(* Logix 5000 AddOnInstructionDefinition export YAI_Assy_155_118_EIP_Hz; software revision 21.03 *)

ADD_ON_INSTRUCTION YAI_Assy_155_118_EIP_Hz   (* revision 1.0, vendor Yaskawa America, Inc. *)
// YAI Assembly 155 and 118
// Help:
// This add-on instruction is for use with input assemblie 166 and output assemblies 116.
// Node_Input_Assy is defined as the node's input assembly integer array.
// Node_Output_Assy is defined as the node's output assembly integer array.
// Torque limit/reference, torque compensation and torque output variables are only available with A1000.
VAR_IN_OUT
   Node_Input_Assy : AB:ETHERNET_MODULE_INT_40Bytes:I:0; {required}   // Input assembly words
   Node_Output_Assy : AB:ETHERNET_MODULE_INT_12Bytes:O:0; {required}   // Output assembly words
END_VAR
VAR_INPUT
   RunFwd : BOOL; {visible}   // Forward run command
   RunRev : BOOL; {visible}   // Reverse run command
   MFI_3 : BOOL; {visible}   // Multi-function input 3
   MFI_4 : BOOL; {visible}   // Multi-function input 4
   MFI_5 : BOOL; {visible}   // Multi-function input 5
   MFI_6 : BOOL; {visible}   // Multi-function input 6
   MFI_7 : BOOL; {visible}   // Multi-function input 7
   MFI_8 : BOOL; {visible}   // Multi-function input 8
   External_Fault : BOOL;   // External fault command (EF0)
   FaultReset : BOOL; {visible}   // Fault reset command
   MFO_1 : BOOL; {visible}   // Multi-function output (M1-M2 for A/P1000, MA/MB/MC for V1000)
   MFO_2 : BOOL; {visible}   // Multi-function output (M3-M4 for A/P1000, P1 for V1000)
   MFO_3 : BOOL; {visible}   // Multi-function output (M5-M6 for A/P1000, P2 for V1000)
   Freq_Ref : REAL; {visible}   // Frequency reference command in Hz (xx.xx resolution)
   Digital_Output_Fault_Enable : BOOL;   // Bit to enable control of fault output relay over the network
END_VAR
VAR_OUTPUT
   Running : BOOL; {access Read Only, visible}   // Drive running forward status bit
   ZSP : BOOL; {access Read Only, visible}   // Drive zero speed status bit
   RunningRev : BOOL; {access Read Only, visible}   // Drive running reverse status bit
   Reset : BOOL; {access Read Only, visible}   // Drive reset command status bit
   At_Speed : BOOL; {access Read Only, visible}   // Drive at commanded speed status bit
   Ready : BOOL; {access Read Only, visible}   // Drive ready status bit
   Alarm : BOOL; {access Read Only, visible}   // Drive alarm status bit
   Faulted : BOOL; {access Read Only, visible}   // Drive faulted status bit
   OPE : BOOL; {access Read Only}   // OPE alarm/fault present
   UV : BOOL; {access Read Only}   // Drive in UV (undervoltage) state status bit
   NetCtrlStatus : BOOL; {access Read Only, visible}   // Drive network run source status bit (1 = source coming from network)
   MFO_1_Status : BOOL; {access Read Only, visible}   // Drive multi-function output 1 (M1-M2 for A/P1000, MA/MB/MC for V1000) status
   MFO_2_Status : BOOL; {access Read Only, visible}   // Drive multi-function output 1 (M3-M4 for A/P1000, P1 for V1000) status
   MFO_3_Status : BOOL; {access Read Only, visible}   // Drive multi-function output 1 (M5-M6 for A/P1000, P2 for V1000) status
   ZSV : BOOL; {access Read Only, visible}   // Drive zero servo completed status bit
   Motor_Speed : REAL; {access Read Only, visible}   // Motor speed in Hz (xx.xx resolution)
   Torque_Actual : REAL; {access Read Only, visible}   // Drive torque output in % (xxx.x resolution)
   PG1_Count : INT; {access Read Only}   // Encoder feedback count
   Freq_Cmd : REAL; {access Read Only, visible}   // Commanded frequency in Hz (xx.xx resolution)
   Output_Freq : REAL; {access Read Only, visible}   // Drive output frequency in Hz (xx.xx resolution)
   Output_Current : REAL; {access Read Only, visible}   // Drive output current in A (xxx.x resolution)
   Analog_Input_1_Level : REAL; {access Read Only}   // Analog input 1 level in % (xxx.x resolution)
   DC_Bus_Volt : INT; {access Read Only, visible}   // DC bus voltage in Vdc (xxx resolution)
   Analog_Input_3_Level : REAL; {access Read Only}   // Analog input 3 level in % (xxx.x resolution)
   Analog_Input_2_Level : REAL; {access Read Only}   // Analog input 2 level in % (xxx.x resolution)
   S1_Status : BOOL; {access Read Only}   // Digital input S1 status
   S2_Status : BOOL; {access Read Only}   // Digital input S2 status
   S3_Status : BOOL; {access Read Only}   // Digital input S3 status
   S4_Status : BOOL; {access Read Only}   // Digital input S4 status
   S5_Status : BOOL; {access Read Only}   // Digital input S5 status
   S6_Status : BOOL; {access Read Only}   // Digital input S6 status
   S7_Status : BOOL; {access Read Only}   // Digital input S7 status
   S8_Status : BOOL; {access Read Only}   // Digital input S8 status
   PG2_Count : INT;   // Encoder 2 feedback count
   UV_Alarm : BOOL; {access Read Only}   // Undervoltage alarm
   OV_Alarm : BOOL; {access Read Only}   // Overvoltage alarm
   OH_Alarm : BOOL; {access Read Only}   // Overheat alarm
   OH2_Alarm : BOOL; {access Read Only}   // Drive overheat alarm
   OL3_Alarm : BOOL; {access Read Only}   // Overtorque detection 1 alarm
   OL4_Alarm : BOOL; {access Read Only}   // Overtorque detection 2 alarm
   EF_Alarm : BOOL; {access Read Only}   // Run command error alarm
   bb_Alarm : BOOL; {access Read Only}   // Baseblock alarm
   EF3_Alarm : BOOL; {access Read Only}   // External fault 3 alarm
   EF4_Alarm : BOOL; {access Read Only}   // External fault 4 alarm
   EF5_Alarm : BOOL; {access Read Only}   // External fault 5 alarm
   EF6_Alarm : BOOL; {access Read Only}   // External fault 6 alarm
   EF7_Alarm : BOOL; {access Read Only}   // External fault 7 alarm
   EF8_Alarm : BOOL; {access Read Only}   // External fault 8 alarm
   FAN_Alarm : BOOL; {access Read Only}   // Cooling fan error alarm
   OS_Alarm : BOOL; {access Read Only}   // Overspeed alarm
   DEV_Alarm : BOOL; {access Read Only}   // Speed deviation alarm
   PGO_Alarm : BOOL; {access Read Only}   // Encoder feedback open alarm
   OPR_Alarm : BOOL; {access Read Only}   // Operator removed alarm
   CE_Alarm : BOOL; {access Read Only}   // Serial communication error alarm
   BUS_Alarm : BOOL; {access Read Only}   // BUS alarm
   CALL_Alarm : BOOL; {access Read Only}   // Serial communication timeout alarm
   OL1_Alarm : BOOL; {access Read Only}   // Motor overload alarm
   OL2_Alarm : BOOL; {access Read Only}   // Drive overload alarm
   EF0_Alarm : BOOL; {access Read Only}   // External fault 0 alarm
   RUN_Alarm : BOOL; {access Read Only}   // Motor 2 run command issued while running alarm
   UL3_Alarm : BOOL; {access Read Only}   // Undertorque detecxtion 1 alarm
   UL4_Alarm : BOOL; {access Read Only}   // Undertorque detection 2 alarm
   SE_Alarm : BOOL; {access Read Only}   // Modbus test failure alarm
   OH3_Alarm : BOOL; {access Read Only}   // Motor overload alarm
   FBL_Alarm : BOOL; {access Read Only}   // PID feedback loss alarm
   FBH_Alarm : BOOL; {access Read Only}   // PID feedback loss alarm
   DNE_Alarm : BOOL; {access Read Only}   // Drive not enabled alarm
END_VAR
VAR_INPUT
   Custom_Out_1 : INT;
   Custom_Out_2 : INT;
   Custom_Out_3 : INT;
   Custom_Out_4 : INT;
END_VAR
VAR
   FRef_Convert : DINT;
   FOut_Convert : REAL;
   FOut_Temp : REAL;
   TRef_Convert : INT;
   TComp_Convert : INT;
   TOut_Convert : REAL;
   TOut_Temp : REAL;
   IOut_Temp : REAL;
   IOut_Convert : REAL;
   AO1_Convert : INT;
   AO2_Convert : INT;
   Motor_Speed_Temp : REAL;
   Motor_Speed_Convert : REAL;
   Freq_Cmd_Temp : REAL;
   Freq_Cmd_Convert : REAL;
   AI1_Temp : REAL;
   AI1_Convert : REAL;
   AI2_Temp : REAL; {access None}
   AI2_Convert : REAL; {access None}
   AI3_Temp : REAL; {access None}
   AI3_Convert : REAL; {access None}
END_VAR

ROUTINE Logic   (* ladder *)
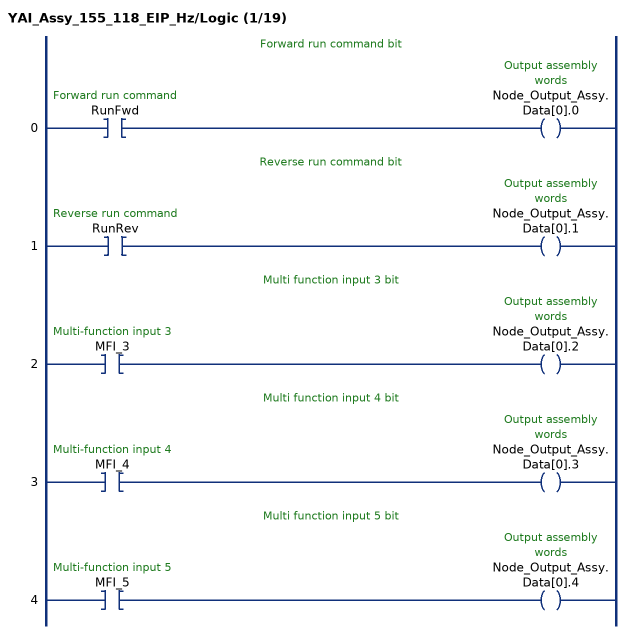
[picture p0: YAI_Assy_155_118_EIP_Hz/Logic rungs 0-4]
   // Forward run command bit
   0: XIC(RunFwd)OTE(Node_Output_Assy.Data[0].0);
   // Reverse run command bit
   1: XIC(RunRev)OTE(Node_Output_Assy.Data[0].1);
   // Multi function input 3 bit
   2: XIC(MFI_3)OTE(Node_Output_Assy.Data[0].2);
   // Multi function input 4 bit
   3: XIC(MFI_4)OTE(Node_Output_Assy.Data[0].3);
   // Multi function input 5 bit
   4: XIC(MFI_5)OTE(Node_Output_Assy.Data[0].4);
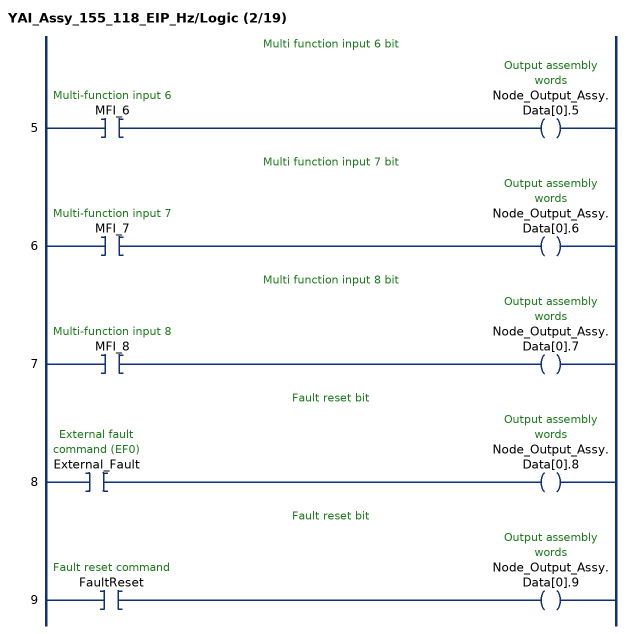
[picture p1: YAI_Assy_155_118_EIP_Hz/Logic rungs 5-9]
   // Multi function input 6 bit
   5: XIC(MFI_6)OTE(Node_Output_Assy.Data[0].5);
   // Multi function input 7 bit
   6: XIC(MFI_7)OTE(Node_Output_Assy.Data[0].6);
   // Multi function input 8 bit
   7: XIC(MFI_8)OTE(Node_Output_Assy.Data[0].7);
   // Fault reset bit
   8: XIC(External_Fault)OTE(Node_Output_Assy.Data[0].8);
   // Fault reset bit
   9: XIC(FaultReset)OTE(Node_Output_Assy.Data[0].9);
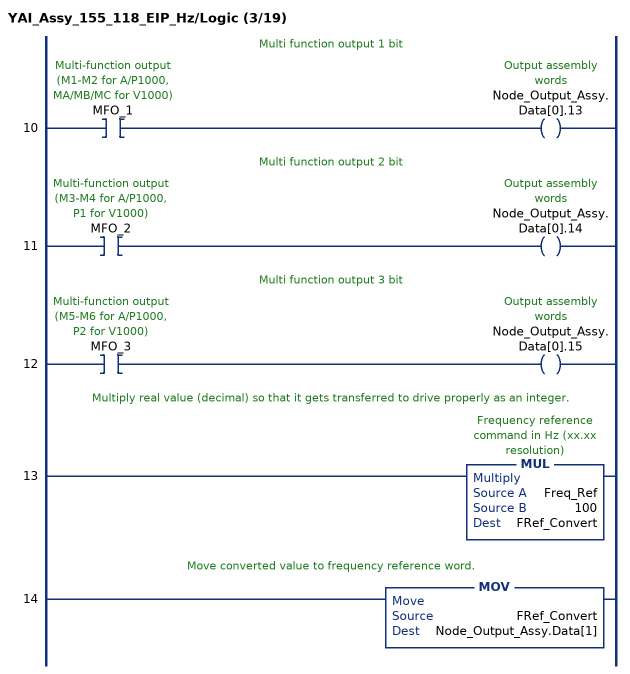
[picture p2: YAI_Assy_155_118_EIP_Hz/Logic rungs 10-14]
   // Multi function output 1 bit
   10: XIC(MFO_1)OTE(Node_Output_Assy.Data[0].13);
   // Multi function output 2 bit
   11: XIC(MFO_2)OTE(Node_Output_Assy.Data[0].14);
   // Multi function output 3 bit
   12: XIC(MFO_3)OTE(Node_Output_Assy.Data[0].15);
   // Multiply real value (decimal) so that it gets transferred to drive properly as an integer.
   13: MUL(Freq_Ref,100,FRef_Convert);
   // Move converted value to frequency reference word.
   14: MOV(FRef_Convert,Node_Output_Assy.Data[1]);
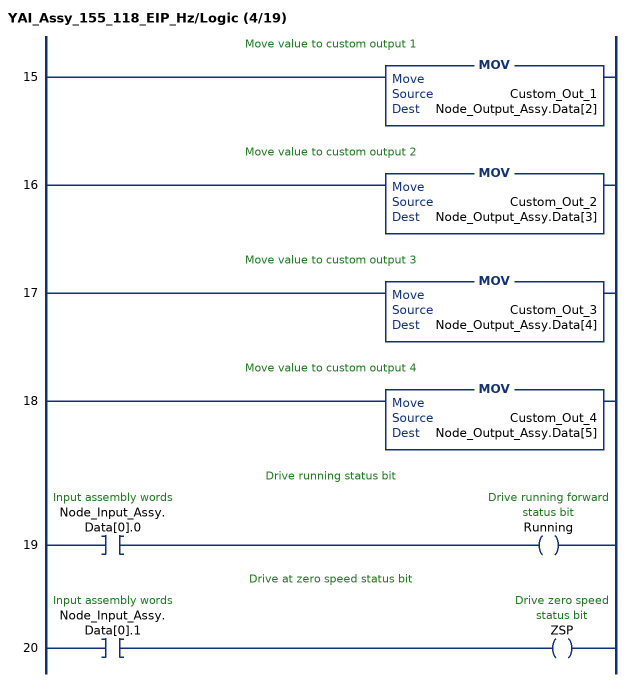
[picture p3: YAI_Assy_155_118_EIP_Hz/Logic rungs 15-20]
   // Move value to custom output 1
   15: MOV(Custom_Out_1,Node_Output_Assy.Data[2]);
   // Move value to custom output 2
   16: MOV(Custom_Out_2,Node_Output_Assy.Data[3]);
   // Move value to custom output 3
   17: MOV(Custom_Out_3,Node_Output_Assy.Data[4]);
   // Move value to custom output 4
   18: MOV(Custom_Out_4,Node_Output_Assy.Data[5]);
   // Drive running status bit
   19: XIC(Node_Input_Assy.Data[0].0)OTE(Running);
   // Drive at zero speed status bit
   20: XIC(Node_Input_Assy.Data[0].1)OTE(ZSP);
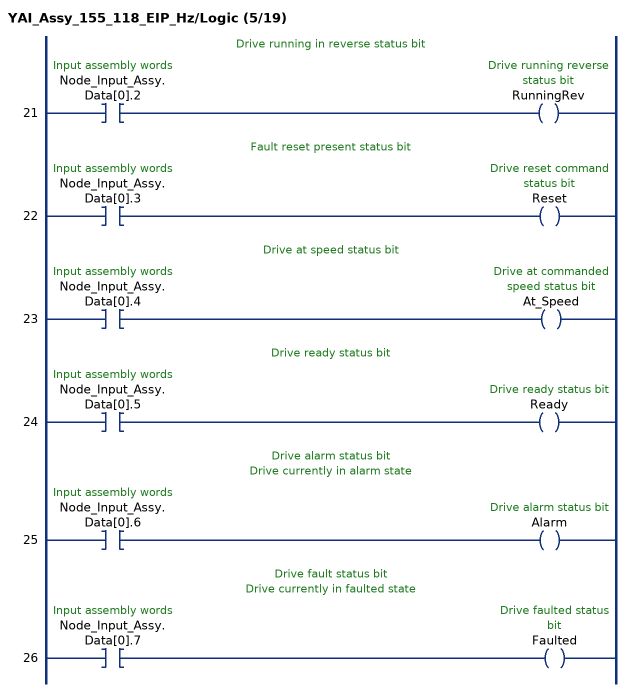
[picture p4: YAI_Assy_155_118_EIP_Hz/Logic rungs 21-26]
   // Drive running in reverse status bit
   21: XIC(Node_Input_Assy.Data[0].2)OTE(RunningRev);
   // Fault reset present status bit
   22: XIC(Node_Input_Assy.Data[0].3)OTE(Reset);
   // Drive at speed status bit
   23: XIC(Node_Input_Assy.Data[0].4)OTE(At_Speed);
   // Drive ready status bit
   24: XIC(Node_Input_Assy.Data[0].5)OTE(Ready);
   // Drive alarm status bit
   // Drive currently in alarm state
   25: XIC(Node_Input_Assy.Data[0].6)OTE(Alarm);
   // Drive fault status bit
   // Drive currently in faulted state
   26: XIC(Node_Input_Assy.Data[0].7)OTE(Faulted);
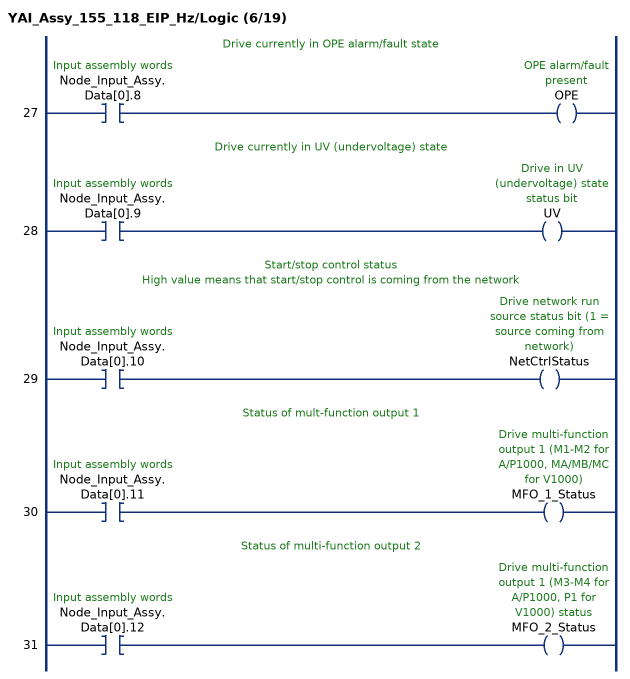
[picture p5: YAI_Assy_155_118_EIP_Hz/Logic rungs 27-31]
   // Drive currently in OPE alarm/fault state
   27: XIC(Node_Input_Assy.Data[0].8)OTE(OPE);
   // Drive currently in UV (undervoltage) state
   28: XIC(Node_Input_Assy.Data[0].9)OTE(UV);
   // Start/stop control status
   // High value means that start/stop control is coming from the network
   29: XIC(Node_Input_Assy.Data[0].10)OTE(NetCtrlStatus);
   // Status of mult-function output 1
   30: XIC(Node_Input_Assy.Data[0].11)OTE(MFO_1_Status);
   // Status of multi-function output 2
   31: XIC(Node_Input_Assy.Data[0].12)OTE(MFO_2_Status);
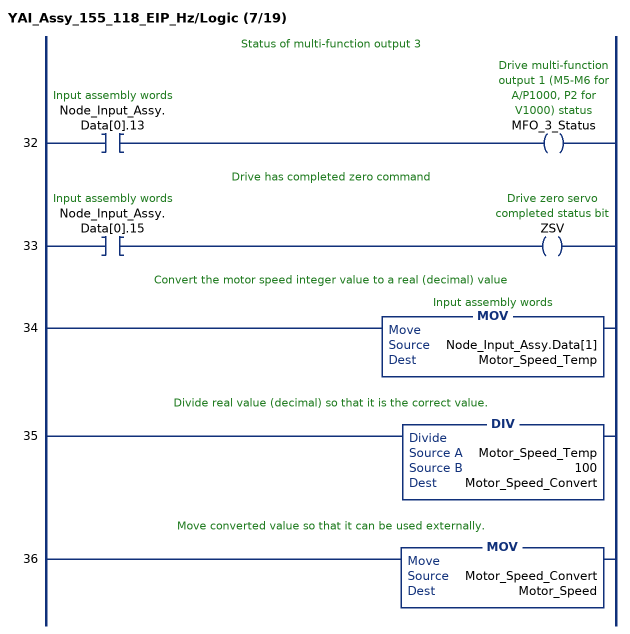
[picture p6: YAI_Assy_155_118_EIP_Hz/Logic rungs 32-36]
   // Status of multi-function output 3
   32: XIC(Node_Input_Assy.Data[0].13)OTE(MFO_3_Status);
   // Drive has completed zero command
   33: XIC(Node_Input_Assy.Data[0].15)OTE(ZSV);
   // Convert the motor speed integer value to a real (decimal) value
   34: MOV(Node_Input_Assy.Data[1],Motor_Speed_Temp);
   // Divide real value (decimal) so that it is the correct value.
   35: DIV(Motor_Speed_Temp,100,Motor_Speed_Convert);
   // Move converted value so that it can be used externally.
   36: MOV(Motor_Speed_Convert,Motor_Speed);
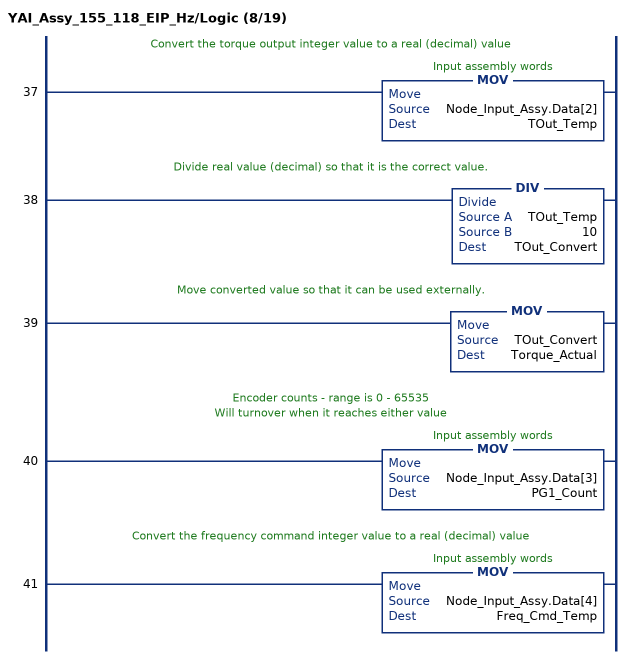
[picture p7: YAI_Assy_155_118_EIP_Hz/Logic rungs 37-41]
   // Convert the torque output integer value to a real (decimal) value
   37: MOV(Node_Input_Assy.Data[2],TOut_Temp);
   // Divide real value (decimal) so that it is the correct value.
   38: DIV(TOut_Temp,10,TOut_Convert);
   // Move converted value so that it can be used externally.
   39: MOV(TOut_Convert,Torque_Actual);
   // Encoder counts - range is 0 - 65535
   // Will turnover when it reaches either value
   40: MOV(Node_Input_Assy.Data[3],PG1_Count);
   // Convert the frequency command integer value to a real (decimal) value
   41: MOV(Node_Input_Assy.Data[4],Freq_Cmd_Temp);
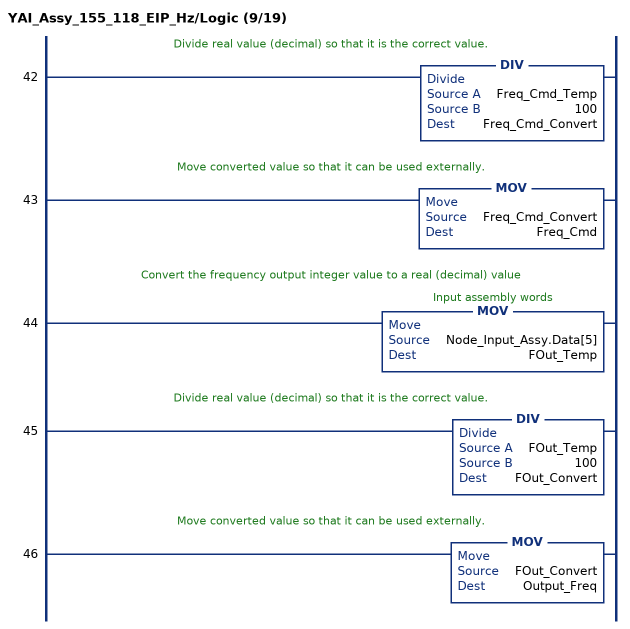
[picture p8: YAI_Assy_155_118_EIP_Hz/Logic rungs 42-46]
   // Divide real value (decimal) so that it is the correct value.
   42: DIV(Freq_Cmd_Temp,100,Freq_Cmd_Convert);
   // Move converted value so that it can be used externally.
   43: MOV(Freq_Cmd_Convert,Freq_Cmd);
   // Convert the frequency output integer value to a real (decimal) value
   44: MOV(Node_Input_Assy.Data[5],FOut_Temp);
   // Divide real value (decimal) so that it is the correct value.
   45: DIV(FOut_Temp,100,FOut_Convert);
   // Move converted value so that it can be used externally.
   46: MOV(FOut_Convert,Output_Freq);
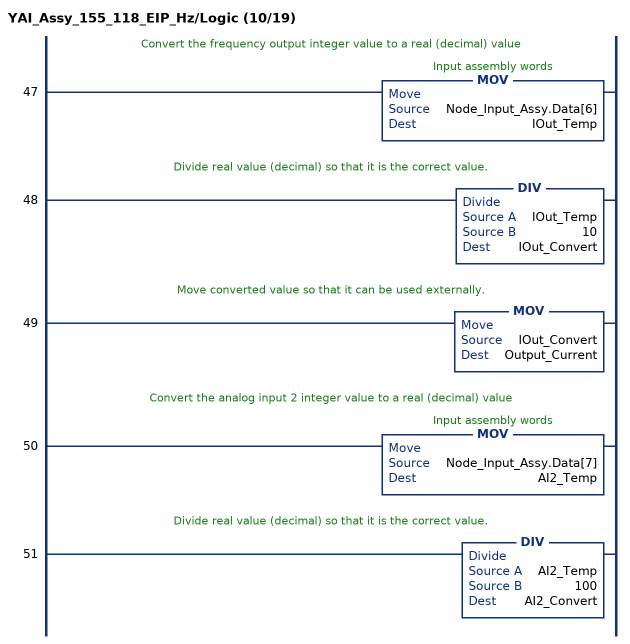
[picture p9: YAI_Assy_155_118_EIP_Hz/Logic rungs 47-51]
   // Convert the frequency output integer value to a real (decimal) value
   47: MOV(Node_Input_Assy.Data[6],IOut_Temp);
   // Divide real value (decimal) so that it is the correct value.
   48: DIV(IOut_Temp,10,IOut_Convert);
   // Move converted value so that it can be used externally.
   49: MOV(IOut_Convert,Output_Current);
   // Convert the analog input 2 integer value to a real (decimal) value
   50: MOV(Node_Input_Assy.Data[7],AI2_Temp);
   // Divide real value (decimal) so that it is the correct value.
   51: DIV(AI2_Temp,100,AI2_Convert);
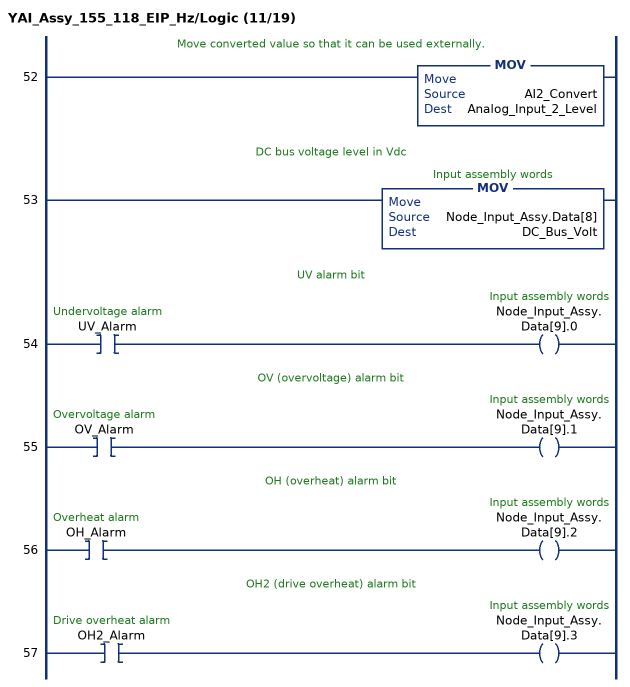
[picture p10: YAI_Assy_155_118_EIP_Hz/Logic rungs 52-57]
   // Move converted value so that it can be used externally.
   52: MOV(AI2_Convert,Analog_Input_2_Level);
   // DC bus voltage level in Vdc
   53: MOV(Node_Input_Assy.Data[8],DC_Bus_Volt);
   // UV alarm bit
   54: XIC(UV_Alarm)OTE(Node_Input_Assy.Data[9].0);
   // OV (overvoltage) alarm bit
   55: XIC(OV_Alarm)OTE(Node_Input_Assy.Data[9].1);
   // OH (overheat) alarm bit
   56: XIC(OH_Alarm)OTE(Node_Input_Assy.Data[9].2);
   // OH2 (drive overheat) alarm bit
   57: XIC(OH2_Alarm)OTE(Node_Input_Assy.Data[9].3);
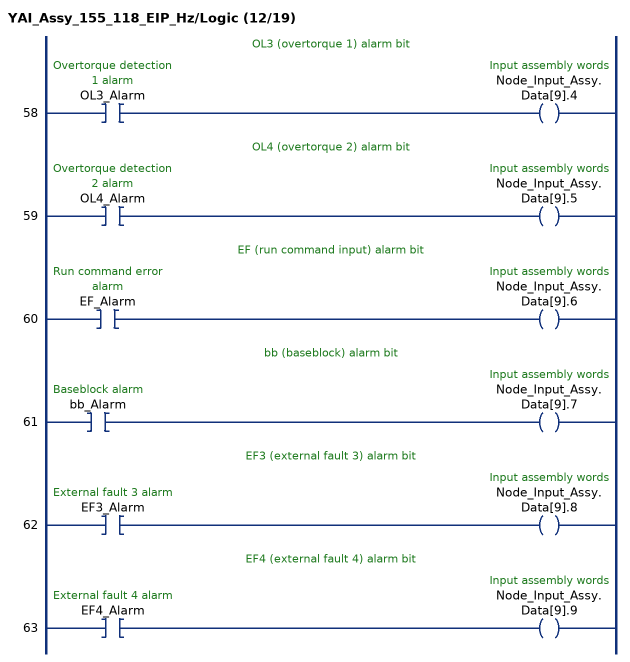
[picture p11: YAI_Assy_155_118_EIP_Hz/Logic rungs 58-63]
   // OL3 (overtorque 1) alarm bit
   58: XIC(OL3_Alarm)OTE(Node_Input_Assy.Data[9].4);
   // OL4 (overtorque 2) alarm bit
   59: XIC(OL4_Alarm)OTE(Node_Input_Assy.Data[9].5);
   // EF (run command input) alarm bit
   60: XIC(EF_Alarm)OTE(Node_Input_Assy.Data[9].6);
   // bb (baseblock) alarm bit
   61: XIC(bb_Alarm)OTE(Node_Input_Assy.Data[9].7);
   // EF3 (external fault 3) alarm bit
   62: XIC(EF3_Alarm)OTE(Node_Input_Assy.Data[9].8);
   // EF4 (external fault 4) alarm bit
   63: XIC(EF4_Alarm)OTE(Node_Input_Assy.Data[9].9);
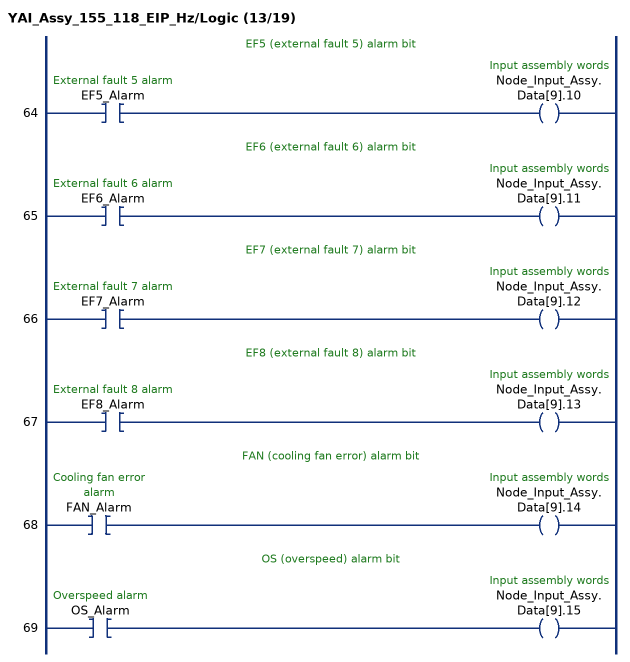
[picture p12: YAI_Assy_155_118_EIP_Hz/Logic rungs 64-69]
   // EF5 (external fault 5) alarm bit
   64: XIC(EF5_Alarm)OTE(Node_Input_Assy.Data[9].10);
   // EF6 (external fault 6) alarm bit
   65: XIC(EF6_Alarm)OTE(Node_Input_Assy.Data[9].11);
   // EF7 (external fault 7) alarm bit
   66: XIC(EF7_Alarm)OTE(Node_Input_Assy.Data[9].12);
   // EF8 (external fault 8) alarm bit
   67: XIC(EF8_Alarm)OTE(Node_Input_Assy.Data[9].13);
   // FAN (cooling fan error) alarm bit
   68: XIC(FAN_Alarm)OTE(Node_Input_Assy.Data[9].14);
   // OS (overspeed) alarm bit
   69: XIC(OS_Alarm)OTE(Node_Input_Assy.Data[9].15);
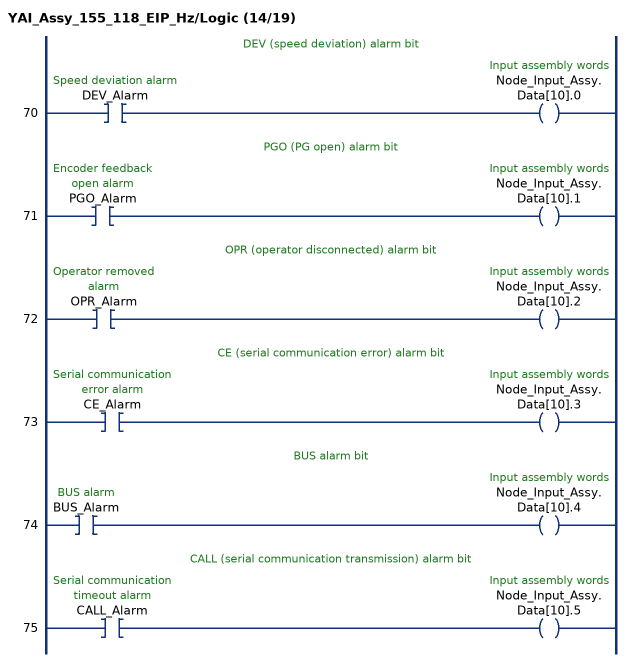
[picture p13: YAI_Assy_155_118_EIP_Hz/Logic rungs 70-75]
   // DEV (speed deviation) alarm bit
   70: XIC(DEV_Alarm)OTE(Node_Input_Assy.Data[10].0);
   // PGO (PG open) alarm bit
   71: XIC(PGO_Alarm)OTE(Node_Input_Assy.Data[10].1);
   // OPR (operator disconnected) alarm bit
   72: XIC(OPR_Alarm)OTE(Node_Input_Assy.Data[10].2);
   // CE (serial communication error) alarm bit
   73: XIC(CE_Alarm)OTE(Node_Input_Assy.Data[10].3);
   // BUS alarm bit
   74: XIC(BUS_Alarm)OTE(Node_Input_Assy.Data[10].4);
   // CALL (serial communication transmission) alarm bit
   75: XIC(CALL_Alarm)OTE(Node_Input_Assy.Data[10].5);
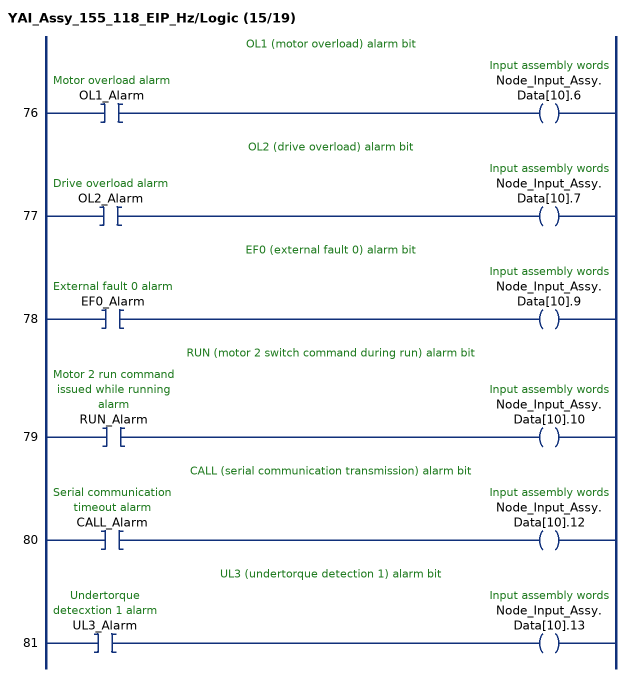
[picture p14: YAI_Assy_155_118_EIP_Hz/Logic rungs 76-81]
   // OL1 (motor overload) alarm bit
   76: XIC(OL1_Alarm)OTE(Node_Input_Assy.Data[10].6);
   // OL2 (drive overload) alarm bit
   77: XIC(OL2_Alarm)OTE(Node_Input_Assy.Data[10].7);
   // EF0 (external fault 0) alarm bit
   78: XIC(EF0_Alarm)OTE(Node_Input_Assy.Data[10].9);
   // RUN (motor 2 switch command during run) alarm bit
   79: XIC(RUN_Alarm)OTE(Node_Input_Assy.Data[10].10);
   // CALL (serial communication transmission) alarm bit
   80: XIC(CALL_Alarm)OTE(Node_Input_Assy.Data[10].12);
   // UL3 (undertorque detection 1) alarm bit
   81: XIC(UL3_Alarm)OTE(Node_Input_Assy.Data[10].13);
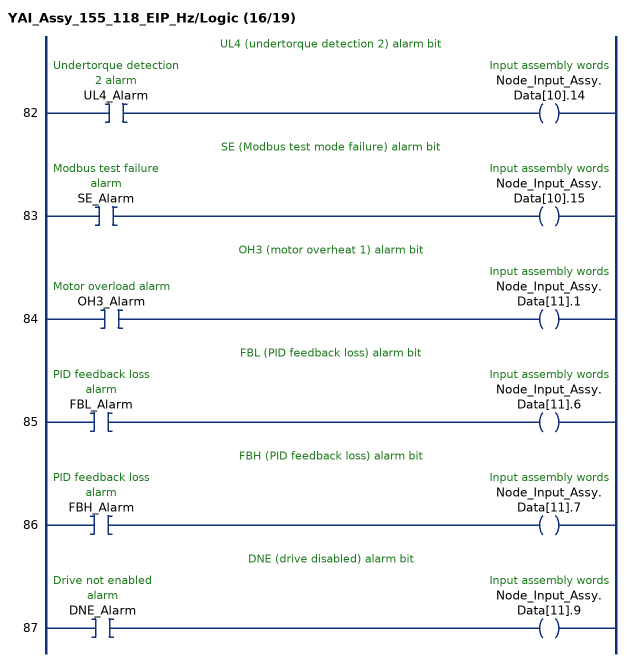
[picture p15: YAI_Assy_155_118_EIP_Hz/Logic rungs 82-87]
   // UL4 (undertorque detection 2) alarm bit
   82: XIC(UL4_Alarm)OTE(Node_Input_Assy.Data[10].14);
   // SE (Modbus test mode failure) alarm bit
   83: XIC(SE_Alarm)OTE(Node_Input_Assy.Data[10].15);
   // OH3 (motor overheat 1) alarm bit
   84: XIC(OH3_Alarm)OTE(Node_Input_Assy.Data[11].1);
   // FBL (PID feedback loss) alarm bit
   85: XIC(FBL_Alarm)OTE(Node_Input_Assy.Data[11].6);
   // FBH (PID feedback loss) alarm bit
   86: XIC(FBH_Alarm)OTE(Node_Input_Assy.Data[11].7);
   // DNE (drive disabled) alarm bit
   87: XIC(DNE_Alarm)OTE(Node_Input_Assy.Data[11].9);
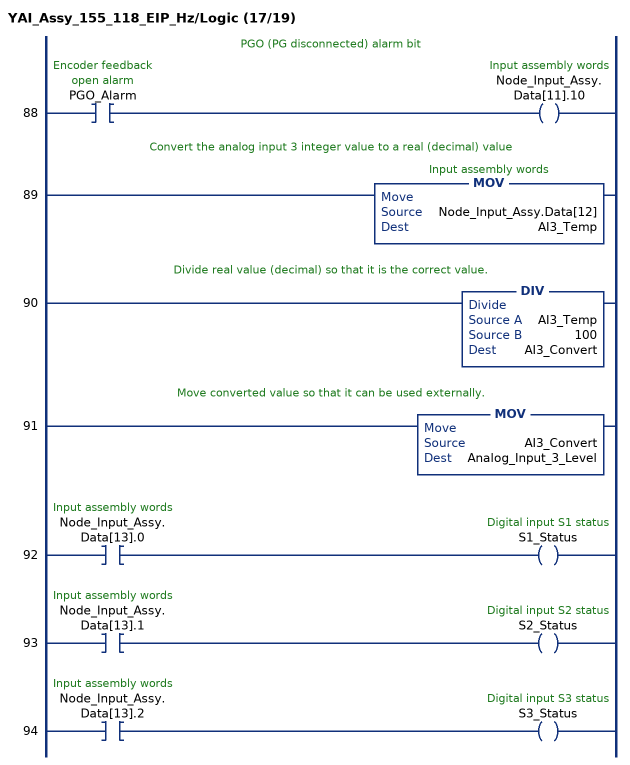
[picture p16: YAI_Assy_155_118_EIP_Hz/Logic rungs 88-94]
   // PGO (PG disconnected) alarm bit
   88: XIC(PGO_Alarm)OTE(Node_Input_Assy.Data[11].10);
   // Convert the analog input 3 integer value to a real (decimal) value
   89: MOV(Node_Input_Assy.Data[12],AI3_Temp);
   // Divide real value (decimal) so that it is the correct value.
   90: DIV(AI3_Temp,100,AI3_Convert);
   // Move converted value so that it can be used externally.
   91: MOV(AI3_Convert,Analog_Input_3_Level);
   92: XIC(Node_Input_Assy.Data[13].0)OTE(S1_Status);
   93: XIC(Node_Input_Assy.Data[13].1)OTE(S2_Status);
   94: XIC(Node_Input_Assy.Data[13].2)OTE(S3_Status);
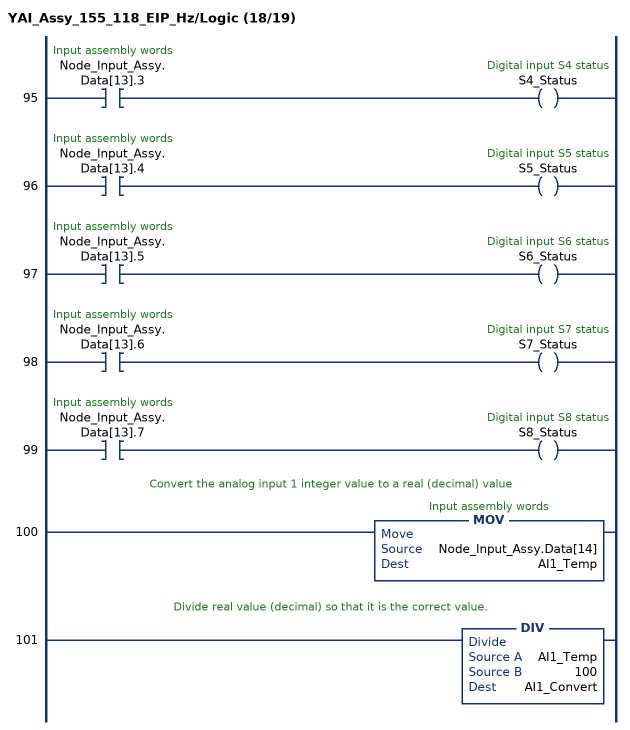
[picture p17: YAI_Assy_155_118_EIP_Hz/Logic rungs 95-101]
   95: XIC(Node_Input_Assy.Data[13].3)OTE(S4_Status);
   96: XIC(Node_Input_Assy.Data[13].4)OTE(S5_Status);
   97: XIC(Node_Input_Assy.Data[13].5)OTE(S6_Status);
   98: XIC(Node_Input_Assy.Data[13].6)OTE(S7_Status);
   99: XIC(Node_Input_Assy.Data[13].7)OTE(S8_Status);
   // Convert the analog input 1 integer value to a real (decimal) value
   100: MOV(Node_Input_Assy.Data[14],AI1_Temp);
   // Divide real value (decimal) so that it is the correct value.
   101: DIV(AI1_Temp,100,AI1_Convert);
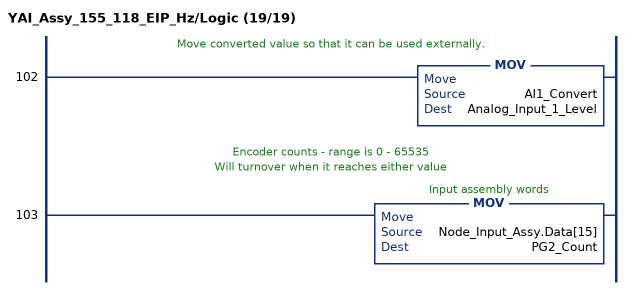
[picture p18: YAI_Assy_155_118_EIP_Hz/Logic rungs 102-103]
   // Move converted value so that it can be used externally.
   102: MOV(AI1_Convert,Analog_Input_1_Level);
   // Encoder counts - range is 0 - 65535
   // Will turnover when it reaches either value
   103: MOV(Node_Input_Assy.Data[15],PG2_Count);
END_ROUTINE
END_ADD_ON_INSTRUCTION
